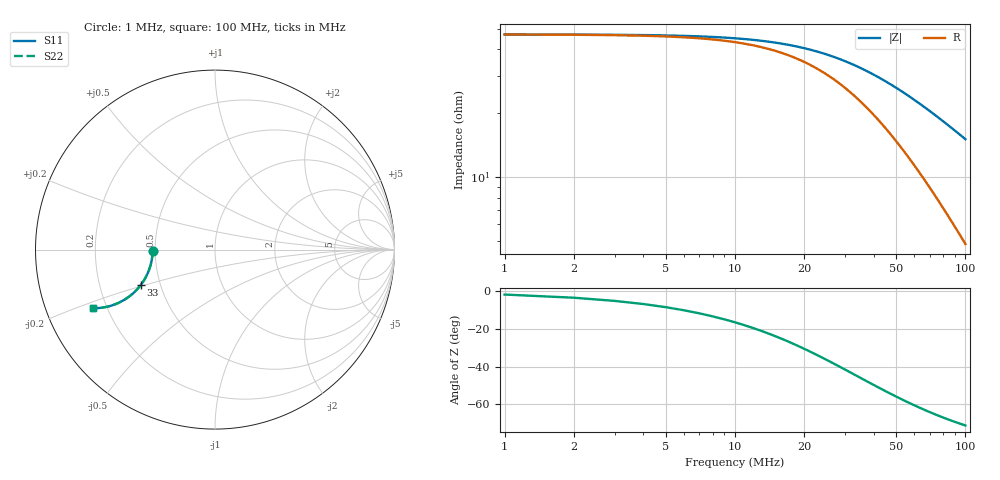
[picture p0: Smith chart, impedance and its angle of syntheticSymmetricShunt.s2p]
# MHz S RI R 50.0000
! SimSmith 18.3b
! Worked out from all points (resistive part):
!   100 points, 1 MHz to 100 MHz, reference 50 ohm
!   read as one part in shunt: R = 47 ohm at 1 MHz
!   S11 on the Smith chart (normalised r, x): 1 MHz: 0.48, -0.01; 33 MHz: 0.39, -0.19; 100 MHz: 0.15, -0.22
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1  -0.3473 -0.00669  0.6527 -0.00669  0.6527 -0.00669  -0.3473 -0.00669
3  -0.3478 -0.0201  0.6522 -0.0201  0.6522 -0.0201  -0.3478 -0.0201
5  -0.3489 -0.0334  0.6511 -0.0334  0.6511 -0.0334  -0.3489 -0.0334
9  -0.3527 -0.0597  0.6473 -0.0597  0.6473 -0.0597  -0.3527 -0.0597
13  -0.3586 -0.0855  0.6414 -0.0855  0.6414 -0.0855  -0.3586 -0.0855
18  -0.3687 -0.1165  0.6313 -0.1165  0.6313 -0.1165  -0.3687 -0.1165
25  -0.3875 -0.157  0.6125 -0.157  0.6125 -0.157  -0.3875 -0.157
29  -0.4003 -0.1783  0.5997 -0.1783  0.5997 -0.1783  -0.4003 -0.1783
33  -0.4143 -0.1982  0.5857 -0.1982  0.5857 -0.1982  -0.4143 -0.1982
34  -0.418 -0.2029  0.582 -0.2029  0.582 -0.2029  -0.418 -0.2029
38  -0.4333 -0.2208  0.5667 -0.2208  0.5667 -0.2208  -0.4333 -0.2208
42  -0.4494 -0.2371  0.5506 -0.2371  0.5506 -0.2371  -0.4494 -0.2371
46  -0.466 -0.2519  0.534 -0.2519  0.534 -0.2519  -0.466 -0.2519
51  -0.4874 -0.2681  0.5126 -0.2681  0.5126 -0.2681  -0.4874 -0.2681
55  -0.5047 -0.2793  0.4953 -0.2793  0.4953 -0.2793  -0.5047 -0.2793
59  -0.5221 -0.2891  0.4779 -0.2891  0.4779 -0.2891  -0.5221 -0.2891
63  -0.5394 -0.2975  0.4606 -0.2975  0.4606 -0.2975  -0.5394 -0.2975
67  -0.5565 -0.3047  0.4435 -0.3047  0.4435 -0.3047  -0.5565 -0.3047
75  -0.5898 -0.3154  0.4102 -0.3154  0.4102 -0.3154  -0.5898 -0.3154
84  -0.6252 -0.3228  0.3748 -0.3228  0.3748 -0.3228  -0.6252 -0.3228
92  -0.6546 -0.3258  0.3454 -0.3258  0.3454 -0.3258  -0.6546 -0.3258
100  -0.6818 -0.3263  0.3182 -0.3263  0.3182 -0.3263  -0.6818 -0.3263
